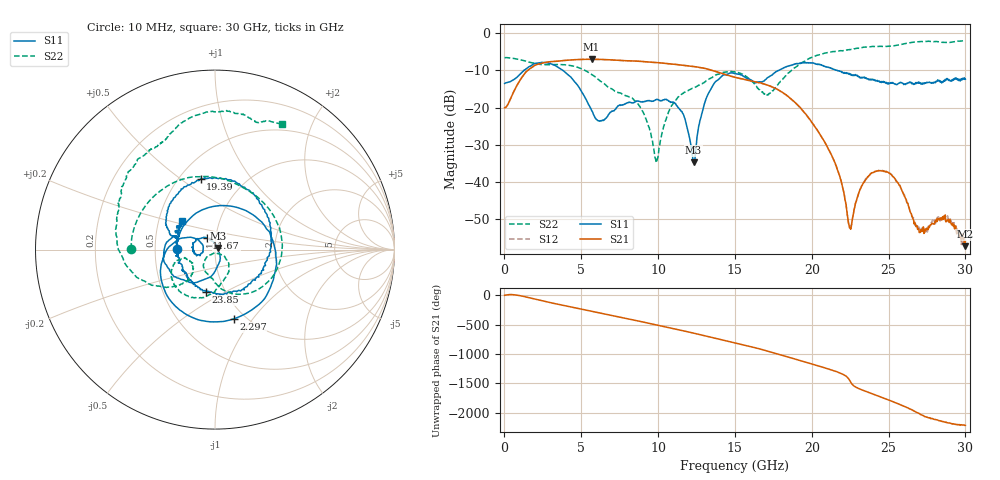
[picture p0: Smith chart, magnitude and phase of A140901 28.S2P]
!  2-Port S-parameters saved by WinCal
! VAR MeasName=S-Parameters (CALIBRATED_DATA) read from VNA (N5244A)
! VAR MeasDate=11/3/2014 9:29:05 AM
! VAR NAME=A140901 28
! VAR FILENAME=A140901 28.S2P
! VAR DATE=11/3/2014 9:29:05 AM
! VAR PHYS_PORTS=1,2
# Hz S RI R 50
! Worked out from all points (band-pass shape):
!   801 points, 10 MHz to 30 GHz, reference 50 ohm
!   highest |S21| = -7.03 dB at 5.671 GHz (marker M1); lowest = -57.2 dB at 29.96 GHz (marker M2)
!   |S21| within 3 dB of the highest: 1.515 GHz to 13.53 GHz (12.02 GHz wide, 160 % of centre)
!   lowest |S11| = -34.8 dB at 12.31 GHz (marker M3), VSWR 1.04, Z = 51.6 + j0.948 ohm
!   |S11| at or under -10 dB: start of sweep to 1.273 GHz; 3.799 GHz to 17.86 GHz (14.06 GHz wide, 130 % of centre); 21.65 GHz to end of sweep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
!   |S22| runs from -34.8 to -2.0 dB; largest |S21 - S12| = 0.0023
!   S11 on the Smith chart (normalised r, x): 10 MHz: 0.65, +0.01; 2.297 GHz: 0.88, -0.81; 11.67 GHz: 0.90, +0.12; 19.39 GHz: 0.63, +0.60; 23.85 GHz: 0.81, -0.41; 30 GHz: 0.66, +0.22
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1e7  -0.2105 0.00513  0.0993 0.00121  0.0997 0.000136  -0.4682 0.00463
9.097e8  0.1282 0.2337  0.2146 -0.00495  0.2143 -0.00477  -0.2799 0.3443
2.296738e9  0.1034 -0.3865  0.0374 -0.3856  0.0373 -0.386  0.1533 0.347
3.796238e9  -0.3017 -0.0956  -0.4182 -0.0775  -0.4188 -0.0769  0.3722 0.054
5.033325e9  -0.1471 0.0681  -0.2406 0.3728  -0.2398 0.3726  0.2491 -0.2167
5.670612e9  -0.0816 0.0418  0.0159 0.445  0.0163 0.4447  0.1244 -0.249
7.470012e9  -0.1022 -0.0326  0.4236 -0.0766  0.4234 -0.0763  -0.0236 -0.1563
1.001916e10  -0.1269 0.0129  -0.3513 -0.1916  -0.351 -0.191  0.0108 -0.0208
1.166861e10  -0.0463 0.0639  -0.1474 0.3382  -0.1479 0.3384  0.0651 -0.1437
1.23059e10  0.0158 0.00918  0.0892 0.3443  0.0897 0.3446  0.0408 -0.1793
1.328058e10  -0.0271 -0.1527  0.3149 0.0842  0.3138 0.0835  -0.00688 -0.2396
1.5005e10  -0.2853 -0.0195  -0.00242 -0.2548  -0.00369 -0.2535  -0.2217 -0.2023
1.71043e10  -0.2382 0.075  -0.1312 0.1524  -0.1305 0.153  -0.1275 -0.0764
1.939104e10  -0.0803 0.3939  0.0659 -0.0644  0.0665 -0.0633  -0.353 -0.1987
2.002832e10  0.0887 0.3887  -0.00352 -0.0621  -0.00274 -0.0622  -0.4518 -0.1371
2.164029e10  0.316 0.0379  -0.011 0.0105  -0.011 0.0106  -0.5472 0.1487
2.246501e10  0.2368 -0.1506  0.00236 -0.000508  0.0024 -0.000375  -0.5387 0.269
2.385205e10  -0.0521 -0.2359  -0.00805 0.0102  -0.00822 0.0101  -0.4342 0.4939
2.501416e10  -0.1637 -0.1269  0.0128 0.00304  0.013 0.00331  -0.3022 0.5941
2.692602e10  -0.2125 0.00102  -0.00209 0.00113  -0.00218 0.00129  -0.0566 0.7623
2.996251e10  -0.1901 0.1445  0.000708 -0.00118  0.00102 -0.00121  0.3732 0.7028
3e10  -0.1822 0.157  0.000847 -0.00136  0.000883 -0.00115  0.3733 0.7006
